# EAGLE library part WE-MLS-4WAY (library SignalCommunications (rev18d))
Multiline EMI Suppression Ferrite Characteristics High impedance common mode inductor with 2x2 windings made by PCB line connection High rated current with typ. 4 A Broadband filtering because of the NiZn-ferrite core RF common mode inductor for 2, 3 or 4 lines in one component Compact size Operating temperature: –25 ºC to +125 ºC Custom designs on request With the appropriate layout (see below) the impedance (i.e. 4 windings) respectively the current (parallel circuit) could be increased Applications Perfect suitable for absorption of common or differential mode interferences in the field of EMC High-current DC output filters of power supplies e.g. battery chargers, industrial power supplies With one turn the component performes like a 3 or 4 times common mode choke for the signal 4-line sensor application Details see: http://katalog.we-online.de/en/pbs/WE-MLS? Updated by Dan Xu 2014-07-08 2014 (C) Wurth Elektronik
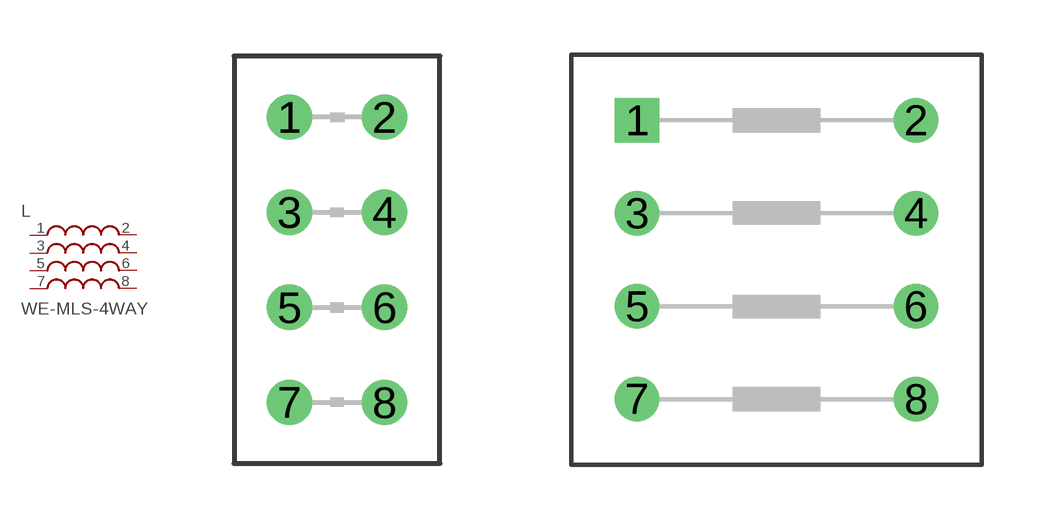
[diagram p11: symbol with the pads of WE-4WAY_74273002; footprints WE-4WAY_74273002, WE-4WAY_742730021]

Designator prefix L

## WE-MLS-4WAY_74273002  [WE-4WAY_74273002]
1  1  pas
2  2  pas
3  3  pas
4  4  pas
5  5  pas
6  6  pas
7  7  pas
8  8  pas

## WE-MLS-4WAY_742730021  [WE-4WAY_742730021]
Pads as for WE-4WAY_74273002

## WE-MLS-4WAY_742730022  [WE-4WAY_742730022]
Pads as for WE-4WAY_74273002

## WE-MLS-4WAY_742730023  [WE-4WAY_742730023]
Pads as for WE-4WAY_74273002

## WE-MLS-4WAY_742730321  [WE-4WAY_742730321]
Pads as for WE-4WAY_74273002

## Footprint WE-4WAY_74273002 (pad centres in mm)
Multiline EMI Suppression Ferrite WE-MLS
drill 0.7: 1 -1.27,3.81; 2 1.27,3.81; 3 -1.27,1.27; 4 1.27,1.27; 5 -1.27,-1.27; 6 1.27,-1.27; 7 -1.27,-3.81; 8 1.27,-3.81

## Footprint WE-4WAY_742730021 (pad centres in mm)
Multiline EMI Suppression Ferrite WE-MLS
drill 0.7 square: 1 -3.81,3.81
drill 0.7: 2 3.81,3.81; 3 -3.81,1.27; 4 3.81,1.27; 5 -3.81,-1.27; 6 3.81,-1.27; 7 -3.81,-3.81; 8 3.81,-3.81

## Footprint WE-4WAY_742730022 (pad centres in mm)
Multiline EMI Suppression Ferrite WE-MLS
drill 0.7: 1 -3.81,3.81; 2 3.81,3.81; 3 -3.81,1.27; 4 3.81,1.27; 5 -3.81,-1.27; 6 3.81,-1.27; 7 -3.81,-3.81; 8 3.81,-3.81

## Footprint WE-4WAY_742730023 (pad centres in mm)
Multiline EMI Suppression Ferrite WE-MLS
drill 0.813: 1 -3.81,3.81; 2 3.81,3.81; 3 -3.81,1.27; 4 3.81,1.27; 5 -3.81,-1.27; 6 3.81,-1.27; 7 -3.81,-3.81; 8 3.81,-3.81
